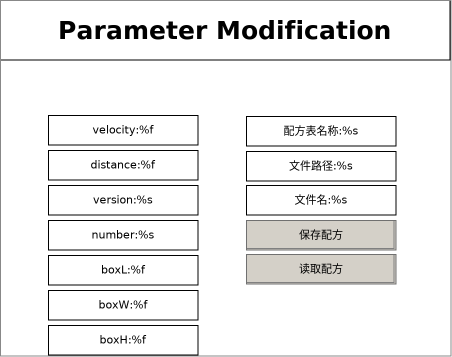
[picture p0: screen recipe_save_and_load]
VISUALIZATION recipe_save_and_load  // 452x357
    Rectangle (0,0 450x60), "Parameter Modification"
    Rectangle (48,115 150x30), "velocity:%f", text variable: velocity
        OnMouseClick: write velocity via Default
    Rectangle (48,150 150x30), "distance:%f", text variable: distance
        OnMouseClick: write the text variable via Default
    Rectangle (48,185 150x30), "version:%s", text variable: version
        OnMouseClick: write the text variable via Default
    Rectangle (48,220 150x30), "number:%s", text variable: number
        OnMouseClick: write the text variable via Default
    Rectangle (246,116 150x30), "配方表名称:%s", text variable: MAIN.recipedefinitionname
        OnMouseClick: write the text variable via Default
    Rectangle (48,255 150x30), "boxL:%f", text variable: boxL
        OnMouseClick: write the text variable via Default
    Rectangle (48,290 150x30), "boxW:%f", text variable: boxW
        OnMouseClick: write the text variable via Default
    Rectangle (48,325 150x30), "boxH:%f", text variable: boxH
        OnMouseClick: write the text variable via Default
    Rectangle (246,151 150x30), "文件路径:%s", text variable: MAIN.sfilepath
        OnMouseClick: write the text variable via Default
    Rectangle (246,185 150x30), "文件名:%s", text variable: MAIN.filename
        OnMouseClick: write the text variable via Default
    Button (246,220 150x30), "保存配方"
        tap MAIN.bsave
    Button (246,254 150x30), "读取配方"
        tap MAIN.bload
END_VISUALIZATION
